VAR_GLOBAL CONSTANT
	(* signal properties *)
	cOversamples 			: UDINT 	:= 10;											// Number of oversamples - 1ms by 10 oversamples => 10 kHz Samplerate 
	cSampleRate     		: LREAL     := 10000.0;										// Samplerate of signal [Hz]

	(* window configuration *)
	cWindowType				: E_CM_WindowType 	:= E_CM_WindowType.eCM_HannWindow;		// window type
	cWindowParameters		: T_CM_WindowParameters := 
							  [0.209671, -0.407331, 0.281225, -0.092669, 0.0091036];	// SFT5M window parameters
	
	(* scaling *)
	cScalingType			: E_CM_ScalingType	:= E_CM_ScalingType.eCM_RootPowerSum;	// scaling of spike energy spectrum
	cTransformToDecibel		: BOOL		:= FALSE;										// transformation to decibel
	
	(* buffer configuration *)
	cWindowLength			: UDINT		:= 800;											// internal buffer size with 50% overlapping
	cOverlap				: UDINT		:= 400;											// size of overlap
	cBufferLength			: UDINT		:= cWindowLength - cOverlap;					// buffer size
	
	(* Spike Energy specific *)
	cDecayTime				: LREAL		:= 1.0 / 107.421875;							// Decay time constant; start with (cWindowLength / cSampleRate)
	cMinFrequency			: LREAL		:= cSampleRate / cWindowLength;				
	
	(* Filter configuration *)
	cLowerFrequencyLimit	: LREAL		:= 1000.0;										// Highpass frequency of bandpass filter [Hz]
	cUpperFrequencyLimit	: LREAL		:= 0.99 * (cSampleRate / 2);					// Lowpass frequency of bandpass filter [Hz]
	cOrder					: UDINT		:= 10;											// Order of bandpass filter in range [1 .. 10]
	
	(* FFT lengths *)
	cFFTLength				: UDINT		:= 1024;										// Length of FFT for internal magnitude spectrum	
	cFFTResult 				: UDINT 	:= cFFTLength/2 + 1;							// Lenght of spectrum (cFFTLength/2+1)
	cResolution 			: LREAL 	:= cSampleRate / cFFTLength;					// Resolution in frequency domain
	
	
END_VAR
